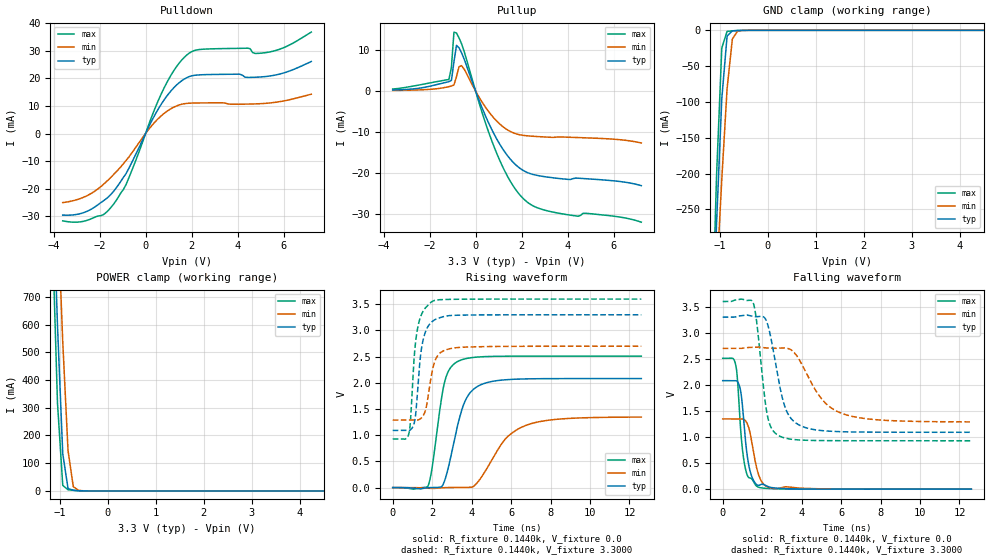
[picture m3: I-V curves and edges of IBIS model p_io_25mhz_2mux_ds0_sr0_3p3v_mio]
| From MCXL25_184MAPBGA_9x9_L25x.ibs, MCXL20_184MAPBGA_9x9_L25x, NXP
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[Model] p_io_25mhz_2mux_ds0_sr0_3p3v_mio
|   Model p_io_25mhz_2mux_ds0_sr0_3p3v_mio
| This model was characterised for following simulation conditions:
| External (pad) voltage:
|   - Typ: 3.3V,   - Min: 2.7V,   - Max: 3.6V
| Library cells for typ/min/max conditions are connected as defined below:
|  pad - External Pad
|  ipp_do_lv - Core Input
|  ipp_obe_lv - Output Buffer Enable
|  IOGC - NC
|  REFH3V3 - REFH3V3
|  REFL3V3 - REFL3V3
|  ZI - NC
|  abut_ncal_vddio[1] - vddio
|  abut_ncal_vddio[2] - vddio
|  abut_ncal_vddio[3] - vssio
|  abut_ncal_vddio[4] - vddio
|  abut_ncal_vddio[5] - vddio
|  abut_ncal_vddio[6] - vssio
|  abut_pcal_vddio[1] - vssio
|  abut_pcal_vddio[2] - vssio
|  abut_pcal_vddio[3] - vddio
|  abut_pcal_vddio[4] - vssio
|  abut_pcal_vddio[5] - vssio
|  abut_pcal_vddio[6] - vddio
|  ipp_do_1p8v - ipp_do_1p8v
|  ipp_dse_lv - 0
|  ipp_eftd_lv - NC
|  ipp_ina_mux_vddio - NC
|  ipp_ina_mux_vddio[0] - NC
|  ipp_ina_mux_vddio[1] - NC
|  ipp_ina_r0_vddio - NC
|  ipp_ina_r0a_vddio - NC
|  ipp_ina_r0b_vddio - NC
|  ipp_ina_r0c_vddio - NC
|  ipp_ina_r0d_vddio - NC
|  ipp_ina_r0e_vddio - NC
|  ipp_ina_r0f_vddio - NC
|  ipp_ina_r300_vddio - NC
|  ipp_ina_r300a_vddio - NC
|  ipp_ina_r300b_vddio - NC
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Model_type I/O
Polarity   Non-Inverting
Enable   Active-High
Vinl =   0.9900V
Vinh =   2.3100V
Vmeas =  1.6500V
Cref =   30.0000pF
Rref =   1.0000M
Vref =   3.3000V
C_comp   1.2811pF   1.2303pF   1.3501pF
|C_comp_pullup   0.5369pF   0.5681pF   0.5156pF
|C_comp_pulldown   0.6705pF   0.7072pF   0.6414pF
[Model Spec]
| variable   typ   min   max
Vinh   2.3100V   1.8900V   2.5200V
Vinl   0.9900V   0.8100V   1.0800V
[Temperature Range]   25.0000   0.1250k   -40.0000
[Voltage Range]   3.3000V   2.7000V   3.6000V
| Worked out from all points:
|   slope of the pulldown table from 0 to 0.495 V, typ, clamps not added: 61.2 ohm
|   slope of the pullup table from 0 to 0.495 V, typ, clamps not added: 71.7 ohm
|   GND clamp passes 1 mA (typ) near -0.74 V on its own axis
|   POWER clamp passes 1 mA (typ) near -0.62 V on its own axis
|   rising waveform, R_fixture 0.1440k, V_fixture 0.0: 20-80 % time 844ps typ, 1.56ns min, 580ps max; typ from 0 V to 2.08 V
|   rising waveform, R_fixture 0.1440k, V_fixture 3.3000: 20-80 % time 369ps typ, 423ps min, 341ps max; typ from 1.09 V to 3.3 V
|   falling waveform, R_fixture 0.1440k, V_fixture 0.0: 20-80 % time 360ps typ, 440ps min, 328ps max; typ from 2.08 V to 0 V
|   falling waveform, R_fixture 0.1440k, V_fixture 3.3000: 20-80 % time 733ps typ, 1.47ns min, 471ps max; typ from 3.3 V to 1.09 V
[Pulldown]
|Voltage   I(typ)   I(min)   I(max)
-3.6V     -29.55mA   -25.02mA   -31.65mA
-2.5V     -28.03mA   -22.34mA   -31.35mA
-1.84V    -24.43mA   -18.49mA   -29.45mA
-1.4V     -21.05mA   -14.95mA   -25.71mA
-850mV    -14.55mA   -9.778mA   -18.51mA
800mV     12.15mA    7.264mA    16.45mA
1.35V     17.61mA    10.02mA    24.32mA
1.9V      20.65mA    11mA       29.17mA
4.43V     20.35mA    10.67mA    30.94mA
4.76V     20.4mA     10.74mA    29.03mA
5.31V     20.76mA    11.01mA    29.46mA
7.2V      26.12mA    14.27mA    36.77mA
[Pullup]
|Voltage   I(typ)   I(min)   I(max)
-3.6V     250.7uA    138.3uA    483.6uA
-1.16V    2.271mA    1.069mA    2.801mA
-1.05V    2.603mA    1.213mA    5.776mA
-940mV    7.093mA    1.465mA    14.38mA
-830mV    11.13mA    3.481mA    14.15mA
-720mV    10.55mA    5.904mA    12.99mA
-610mV    9.336mA    6.198mA    11.54mA
820mV     -10.68mA   -6.749mA   -13.84mA
1.48V     -16.43mA   -9.783mA   -21.75mA
2.03V     -19.25mA   -10.79mA   -26.01mA
3.35V     -21.16mA   -11.31mA   -29.53mA
7.2V      -23.09mA   -12.68mA   -32mA
[GND_clamp]
|Voltage   I(typ)   I(min)   I(max)
-3.6V     -5.309A    -4.128A    -6.876A
-1.18V    -466mA     -495.4mA   -458.9mA
-1.07V    -271.1mA   -348.5mA   -204.6mA
-960mV    -95.65mA   -208mA     -24.74mA
-850mV    -8.096mA   -81.85mA   -1.474mA
-740mV    -719.7uA   -12.14mA   -719.4uA
-630mV    -272.5uA   -923.5uA   -301.7uA
-300mV    -385.6nA   -2.502uA   -74.93nA
7.2V      0A         0A         0A
[POWER_clamp]
|Voltage   I(typ)   I(min)   I(max)
-3.6V     14.48A     12.95A     16.35A
-1.16V    1.177A     1.535A     951.2mA
-1.05V    598.4mA    1.032A     318mA
-940mV    134.2mA    537.3mA    20.02mA
-830mV    8.708mA    145.4mA    4.242mA
-720mV    2.127mA    15.38mA    2.218mA
-610mV    847.4uA    1.853mA    834.1uA
7.2V      0A         0A         0A
[Ramp]
| variable   typ   min   max
dV/dt_r  1.2492/0.8441n   0.8078/1.5632n   1.5061/0.5798n
dV/dt_f  1.3253/0.7333n   0.8457/1.4717n   1.6029/0.4715n
R_load = 0.1440k
[Rising Waveform]
R_fixture= 0.1440k
V_fixture= 0.0
V_fixture_min= 0.0
V_fixture_max= 0.0
|time   V(typ)   V(min)   V(max)
0s        4.603nV    154.1nV    15.8nV
1.784ns   -2.583mV   -13.13mV   27.47mV
1.988ns   647.7uV    -16.58mV   357mV
2.603ns   102.3mV    -809.1uV   1.973V
3.264ns   1.149V     1.101mV    2.402V
3.824ns   1.76V      3.183mV    2.471V
4.799ns   2.007V     380.9mV    2.503V
5.757ns   2.06V      947.3mV    2.509V
6.827ns   2.076V     1.198V     2.51V
12.6ns    2.082V     1.346V     2.51V
[Rising Waveform]
R_fixture= 0.1440k
V_fixture= 3.3000
V_fixture_min= 2.7000
V_fixture_max= 3.6000
|time   V(typ)   V(min)   V(max)
0s        1.091V     1.288V     928.6mV
808.6ps   1.091V     1.288V     1.015V
902.3ps   1.103V     1.288V     1.283V
1.055ns   1.19V      1.289V     2.311V
1.225ns   1.663V     1.289V     2.964V
1.489ns   2.722V     1.344V     3.331V
2.015ns   3.175V     2.246V     3.558V
2.365ns   3.241V     2.558V     3.587V
3.24ns    3.291V     2.672V     3.596V
12.6ns    3.3V       2.7V       3.6V
[Falling Waveform]
R_fixture= 0.1440k
V_fixture= 0.0
V_fixture_min= 0.0
V_fixture_max= 0.0
|time   V(typ)   V(min)   V(max)
0s        2.082V     1.348V     2.51V
616.7ps   2.083V     1.348V     2.443V
726.5ps   2.071V     1.348V     2.202V
836.5ps   1.995V     1.348V     1.571V
981.1ps   1.676V     1.349V     829.3mV
1.162ns   900.2mV    1.309V     374mV
1.408ns   317.4mV    1.038V     214.6mV
1.786ns   75.23mV    316.7mV    41.7mV
2.634ns   22.76mV    12.15mV    7.932mV
12.6ns    198.7nV    13.86uV    45.49nV
[Falling Waveform]
R_fixture= 0.1440k
V_fixture= 3.3000
V_fixture_min= 2.7000
V_fixture_max= 3.6000
|time   V(typ)   V(min)   V(max)
0s        3.3V       2.7V       3.6V
1.546ns   3.315V     2.723V     3.575V
1.72ns    3.308V     2.726V     3.217V
2.266ns   3.176V     2.707V     1.408V
2.856ns   2.037V     2.706V     1.023V
3.207ns   1.524V     2.706V     975.6mV
3.648ns   1.287V     2.61V      950.5mV
5.01ns    1.124V     1.735V     932mV
6.047ns   1.102V     1.452V     929.7mV
12.6ns    1.091V     1.29V      928.6mV
